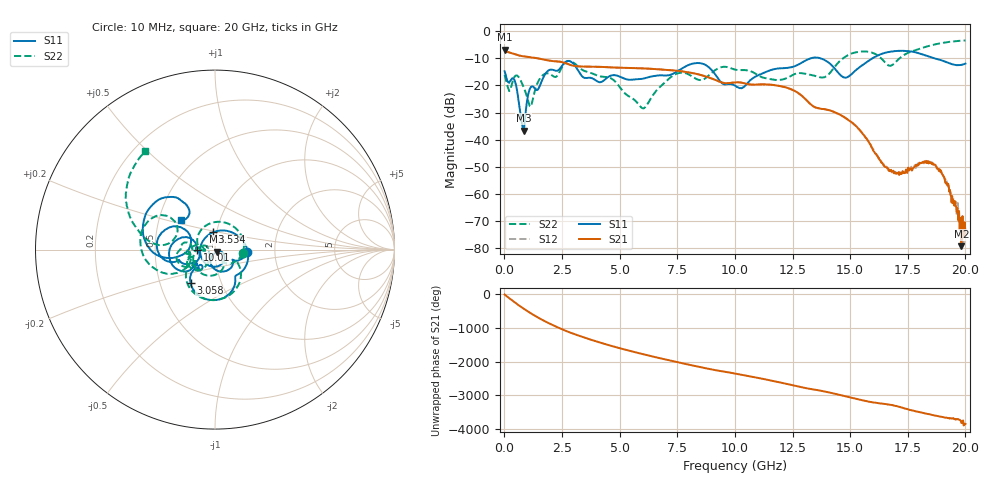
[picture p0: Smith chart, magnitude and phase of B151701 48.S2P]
!  2-Port S-parameters saved by WinCal
! VAR MeasName=S-Parameters (CALIBRATED_DATA) read from VNA (N5244A)
! VAR MeasDate=2015-12-24 19:15:07
! VAR NAME=B151701 48
! VAR FILENAME=B151701 48.S2P
! VAR DATE=2015-12-24 19:15:07
! VAR PHYS_PORTS=1,3
# Hz S DB R 50
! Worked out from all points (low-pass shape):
!   801 points, 10 MHz to 20 GHz, reference 50 ohm
!   highest |S21| = -6.89 dB at 10 MHz (marker M1); lowest = -79.2 dB at 19.83 GHz (marker M2)
!   |S21| within 3 dB of the highest: start of sweep to 1.353 GHz
!   lowest |S11| = -36.6 dB at 834.6 MHz (marker M3), VSWR 1.03, Z = 50.9 - j1.22 ohm
!   |S11| at or under -10 dB: start of sweep to 13.31 GHz; 13.7 GHz to 15.98 GHz (2.278 GHz wide, 15.4 % of centre); 18.64 GHz to end of sweep
!   |S22| runs from -28.5 to -3.5 dB; largest |S21 - S12| = 0.0011
!   S11 on the Smith chart (normalised r, x): 10 MHz: 1.44, -0.04; 1.534 GHz: 0.96, +0.19; 3.058 GHz: 0.71, -0.28; 10.01 GHz: 0.82, -0.00; 20 GHz: 0.65, +0.22
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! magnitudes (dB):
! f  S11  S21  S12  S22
! 10 MHz  -14.8  -6.9  -6.9  -16.2
! 209.9 MHz  -19.0  -7.9  -7.9  -22.1
! 434.8 MHz  -18.0  -8.4  -8.4  -16.9
! 834.6 MHz  -36.6  -9.3  -9.3  -20.7
! 1.134 GHz  -20.8  -9.6  -9.6  -27.9
! 1.534 GHz  -20.2  -10.2  -10.2  -17.6
! 1.934 GHz  -14.4  -10.9  -10.9  -15.7
! 3.058 GHz  -12.7  -12.9  -12.9  -12.0
! 3.358 GHz  -16.5  -13.1  -13.1  -14.2
! 5.982 GHz  -17.6  -13.7  -13.7  -28.4
! 6.682 GHz  -16.4  -14.1  -14.1  -21.1
! 7.581 GHz  -14.4  -14.7  -14.7  -15.4
! 8.481 GHz  -11.8  -16.1  -16.1  -18.0
! 10.01 GHz  -20.1  -18.9  -18.9  -14.2
! 12.25 GHz  -13.6  -20.8  -20.8  -17.3
! 13.35 GHz  -9.9  -27.4  -27.4  -16.2
! 14.8 GHz  -17.1  -32.1  -31.9  -9.4
! 16.68 GHz  -7.7  -51.4  -50.8  -12.7
! 18.63 GHz  -10.0  -49.0  -49.2  -5.0
! 19.58 GHz  -12.5  -64.2  -63.3  -3.7
! 19.83 GHz  -12.5  -79.2  -72.4  -3.6
! 20 GHz  -12.0  -74.5  -73.2  -3.5
